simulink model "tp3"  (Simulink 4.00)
settings: Solver=ode45  StartTime=0.0  StopTime=tfinal  RelTol=1e-3
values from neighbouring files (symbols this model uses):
  m = 4    [demo1dat.m]    (also in demo2dat.m = 3; essai1dat.m; essai2dat.m = 6; mynlcmpc.m = mp(1:max(size(mp))-1))
  model = tfd2step(1.6,delt,1,g)    [essai2dat.m]    (also in mynlcmpc.m = modelpd(:,1:nu); mynlcmpc2.m = modelpd(:,1:nu); mynlcmpc3.m = modelpd(:,1:nu); scrtp1.m = tfd2step(tfinal,Ts,1,g))
  p = 10    [demo1dat.m]    (also in demo2dat.m; essai1dat.m; essai2dat.m; mynlcmpc.m = mp(max(size(mp))))
  Ts = [tsamp 0]    [mynlcmpc.m]    (also in mynlcmpc2.m; mynlcmpc3.m; scrtp1.m = 0.1; Smpc.m)
  ulim = [-5 40 3]    [essai2dat.m]    (also in mynlcmpc.m = [-inf*ones(1,nu) inf*ones(1,nu) 1e6*ones(1,nu)]; mynlcmpc2.m = [-inf*ones(1,nu) inf*ones(1,nu) 1e6*ones(1,nu)]; mynlcmpc3.m = [-inf*ones(1,nu) inf*ones(1,nu) 1e6*ones(1,nu)]; pmlin.m = [-10*[1 1] 10*[1 1] 2*[1 1]])
  uwt = [0 0]    [demo1dat.m]    (also in demo2dat.m = 0.6*[1 1]; essai1dat.m; essai2dat.m = 1; mynlcmpc.m = ryuwt(:,2*ny+1:2*ny+nu))
  ylim = [-40 40]    [essai2dat.m]    (also in mynlcmpc.m = [ylim; ylim(N,:)]; mynlcmpc2.m = [ylim; ylim(N,:)]; mynlcmpc3.m = [ylim; ylim(N,:)]; pmlin.m = [])
  ywt = [1 1]    [demo1dat.m]    (also in demo2dat.m = [0.2,0,1]; essai1dat.m; essai2dat.m = 1; mynlcmpc.m = ryuwt(:,ny+1:2*ny))

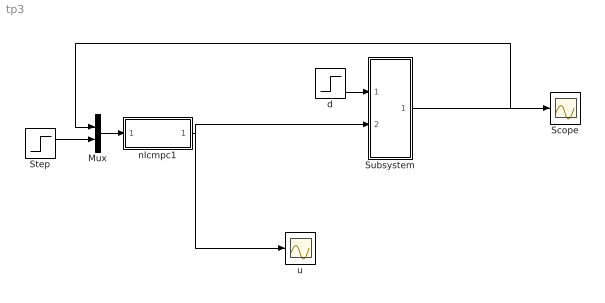
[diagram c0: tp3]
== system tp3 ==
  Mux : Mux  Inputs=2
  Scope : Scope
  Step : Step  Time=1  Before=0  After=1  SampleTime=0
  Subsystem : Subsystem
  d : Step  Time=1  Before=0  After=1  SampleTime=0
  nlcmpc1 : Subsystem  AncestorBlock=nlmpclib/nlcmpc  mask(myCMPC-SIMULINK){modelpd=[model []], yuwt=[ywt uwt], mp=[m p], yulim=[ylim ulim], tfilter=[], ud0=[0 []]}
      mask help: Masked MATLAB function block calls nlcmpc, links CMPC and SIMULINK.
  u : Scope
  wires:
  nlcmpc1/1(Out1) -> u/1, Subsystem/2(In2)
  Mux/1 -> nlcmpc1/1(In1)
  Step/1 -> Mux/2
  d/1 -> Subsystem/1(In1)
  Subsystem/1(Out1) -> Mux/1, Scope/1

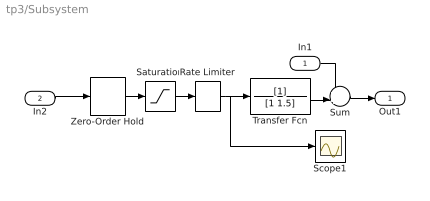
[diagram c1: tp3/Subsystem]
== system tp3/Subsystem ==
  In1 : Inport  Port=1  LatchInput=off
  In2 : Inport  Port=2  LatchInput=off
  Rate Limiter : RateLimiter  RisingSlewLimit=1/Ts  FallingSlewLimit=-1/Ts
  Saturation : Saturate  UpperLimit=2  LowerLimit=-2  LinearizeAsGain=on
  Scope1 : Scope
  Sum : Sum  Inputs=++|  SaturateOnIntegerOverflow=on
  Transfer Fcn : TransferFcn  Numerator=[1]  Denominator=[1 1.5]  AbsoluteTolerance=auto  Realization=auto
  Zero-Order Hold : ZeroOrderHold  SampleTime=Ts
  Out1 : Outport  Port=1
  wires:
  Zero-Order Hold/1 -> Saturation/1
  Saturation/1 -> Rate Limiter/1
  Rate Limiter/1 -> Transfer Fcn/1, Scope1/1
  Transfer Fcn/1 -> Sum/2
  In2/1 -> Zero-Order Hold/1
  In1/1 -> Sum/1
  Sum/1 -> Out1/1

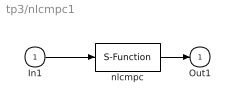
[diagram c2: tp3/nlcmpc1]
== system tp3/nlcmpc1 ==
  In1 : Inport  Port=1  LatchInput=off
  nlcmpc : S-Function  FunctionName=mynlcmpc3  Parameters=modelpd,mp,tfilter,yuwt,ud0,yulim  PortCounts=[]  SFunctionModules=''
  Out1 : Outport  Port=1  InitialOutput=0
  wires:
  In1/1 -> nlcmpc/1
  nlcmpc/1 -> Out1/1
